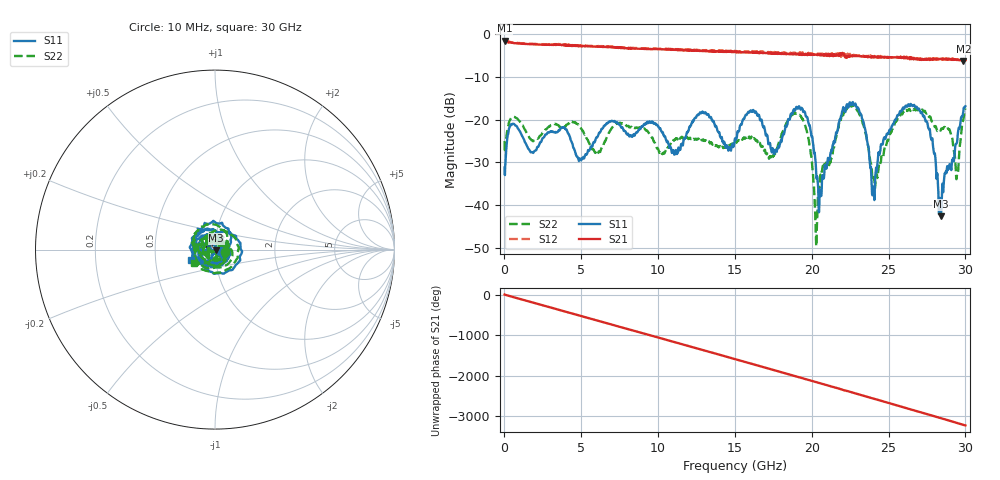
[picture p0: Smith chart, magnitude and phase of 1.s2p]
!Agilent Technologies,E8364B,US42250130,A.04.87.01
!Agilent E8364B: A.04.87.01
!Date: Monday, February 07, 2022 23:47:16
!Correction: S11(Full 2 Port SOLT,1,2) S21(Full 2 Port SOLT,1,2) S12(Full 2 Port SOLT,1,2) S22(Full 2 Port SOLT,1,2)
!S2P File: Measurements: S11, S21, S12, S22:
# Hz S  dB  R 50
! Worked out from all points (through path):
!   1601 points, 10 MHz to 30 GHz, reference 50 ohm
!   highest |S21| = -1.53 dB at 28.74 MHz (marker M1); lowest = -6.3 dB at 29.87 GHz (marker M2)
!   group delay of S21, straight-line fit = 298 ps
!   lowest |S11| = -42.6 dB at 28.41 GHz (marker M3), VSWR 1.01, Z = 50.7 - j0.287 ohm
!   |S11| at or under -10 dB: start of sweep to end of sweep
!   |S22| runs from -49.6 to -16.5 dB; largest |S21 - S12| = 0.076
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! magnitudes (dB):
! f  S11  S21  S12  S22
! 10 MHz  -31.2  -1.5  -1.5  -25.0
! 28.74 MHz  -33.0  -1.5  -1.5  -27.7
! 553.6 MHz  -21.0  -2.0  -1.9  -19.4
! 5.015 GHz  -29.4  -2.7  -2.6  -22.2
! 6.851 GHz  -20.4  -3.0  -3.0  -22.7
! 10.02 GHz  -21.7  -3.5  -3.4  -27.0
! 15.01 GHz  -24.4  -4.1  -4.1  -25.4
! 16.13 GHz  -18.0  -4.2  -3.9  -24.3
! 17.37 GHz  -27.1  -4.5  -4.4  -29.2
! 19.02 GHz  -17.0  -4.7  -4.3  -18.5
! 20.01 GHz  -23.9  -4.7  -4.5  -29.9
! 20.27 GHz  -31.3  -4.8  -4.6  -47.6
! 20.52 GHz  -36.7  -4.9  -4.6  -35.4
! 22.39 GHz  -17.1  -5.1  -4.8  -16.8
! 23.31 GHz  -20.0  -5.2  -5.1  -20.8
! 24 GHz  -36.3  -5.3  -5.2  -33.6
! 25.01 GHz  -23.0  -5.5  -5.4  -24.3
! 27.08 GHz  -18.2  -5.7  -5.9  -17.9
! 28.41 GHz  -42.6  -5.8  -5.8  -22.5
! 29.44 GHz  -25.5  -6.0  -6.0  -33.5
! 29.87 GHz  -18.0  -6.3  -5.8  -20.0
! 30 GHz  -16.9  -6.1  -6.2  -17.3
